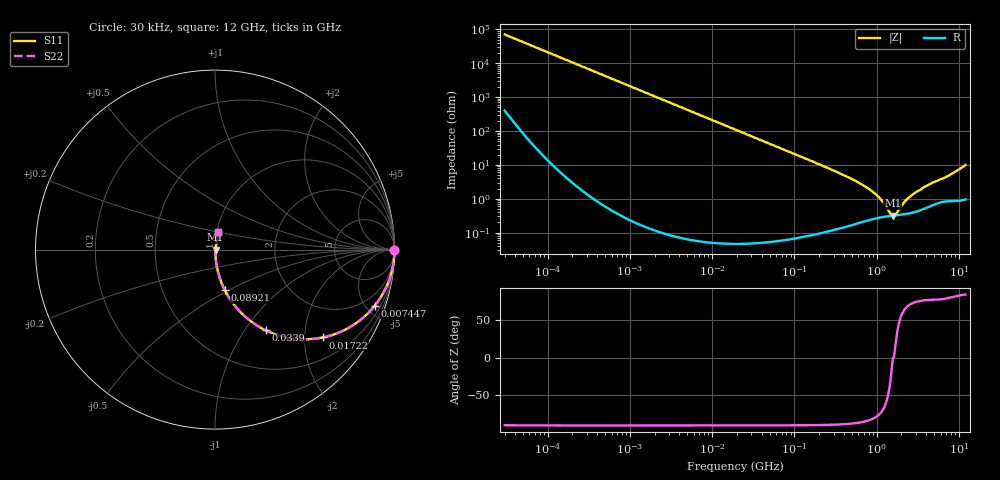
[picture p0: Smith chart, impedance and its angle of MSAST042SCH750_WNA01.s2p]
! MSAST042SCH750_WNA01  S-PARAMETER MODEL  ( General Type )
! Model Generated by TAIYO YUDEN Corporation (http://www.ty-top.com)
! Version 1.0
! TAIYO YUDEN Control No. 150820
! Copyright(c) 2015 TAIYO YUDEN CO.,LTD. All Rights Reserved.
! Product Description (link to TY-COMPAS)
! https://ds.yuden.co.jp/TYCOMPAS/or/detail?pn=MSAST042SCH750JWNA01&u=M
! Products Name : Multilayer Ceramic Capacitors
! Characteristics :
!  Capacitance : 75 pF , Rated Voltage : 25V , TCC : CH / C0H
!  Case Size : 0.4 x 0.2 / 0.016 x 0.008 [mm/inch] , Thickness : 0.2 / 0.008 [mm/inch]
!  (Conditions: Temperature = 25 degC , DC Bias Current/Voltage = 0A / 0V)
! External Node Assignments :
!  1  o---| |---o  2
! GND o---------o GND
! Frequency Range : 0.03MHz  -  12000MHz  [ 401 STEP ]
# MHz S RI R 50
! Freq[MHz].  S11 Real  S11 Imag  S21 Real  S21 Imag  S12 Real  S12 Imag  S22 Real  S22 Imag
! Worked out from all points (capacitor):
!   401 points, 30 kHz to 12 GHz, reference 50 ohm
!   read as one part in series: C = 75 pF near 32 kHz
!   lowest |Z| = 314 mohm at 1.573 GHz (marker M1)
!   series resonance near 1.581 GHz, so ESL is about 140 pH
!   S11 on the Smith chart (normalised r, x): 30 kHz: open; 7.447 MHz: 1.00, -5.70; 17.22 MHz: 1.00, -2.46; 33.9 MHz: 1.00, -1.25; 89.21 MHz: 1.00, -0.47; 12 GHz: 1.02, +0.20
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0.03  1 -0.00141  1e-05 0.00141  1e-05 0.00141  1 -0.00141
0.260295  0.9998 -0.0123  0.000153 0.0123  0.000153 0.0123  0.9998 -0.0123
2.258455  0.9888 -0.1052  0.0112 0.1052  0.0112 0.1052  0.9888 -0.1052
7.447352  0.8903 -0.3124  0.1097 0.3124  0.1097 0.3124  0.8903 -0.3124
11.3258  0.7782 -0.4153  0.2218 0.4153  0.2218 0.4153  0.7782 -0.4153
17.22407  0.6027 -0.4891  0.3973 0.4891  0.3973 0.4891  0.6027 -0.4891
18.97367  0.5556 -0.4967  0.4444 0.4967  0.4444 0.4967  0.5556 -0.4967
33.90345  0.2815 -0.4493  0.7185 0.4493  0.7185 0.4493  0.2815 -0.4493
53.24956  0.1371 -0.3433  0.8629 0.3433  0.8629 0.3433  0.1371 -0.3433
89.2069  0.0538 -0.2242  0.9462 0.2242  0.9462 0.2242  0.0538 -0.2242
164.6252  0.0168 -0.1252  0.9832 0.1252  0.9832 0.1252  0.0168 -0.1252
419.4166  0.00367 -0.0468  0.9963 0.0468  0.9963 0.0468  0.00367 -0.0468
749.4426  0.0027 -0.0218  0.9973 0.0218  0.9973 0.0218  0.0027 -0.0218
1068.55  0.00286 -0.0106  0.9971 0.0106  0.9971 0.0106  0.00286 -0.0106
1215.67  0.00296 -0.00699  0.997 0.00699  0.997 0.00699  0.00296 -0.00699
1428.372  0.00308 -0.0026  0.9969 0.0026  0.9969 0.0026  0.00308 -0.0026
1573.464  0.00313 -9.94e-06  0.9969 9.94e-06  0.9969 9.94e-06  0.00313 -9.94e-06
1733.294  0.00324 0.00155  0.9968 -0.00155  0.9968 -0.00155  0.00324 0.00155
2243.435  0.00359 0.0079  0.9964 -0.0079  0.9964 -0.0079  0.00359 0.0079
2903.719  0.00422 0.0141  0.9958 -0.0141  0.9958 -0.0141  0.00422 0.0141
7640.278  0.0107 0.0478  0.9893 -0.0478  0.9893 -0.0478  0.0107 0.0478
12000  0.0189 0.0959  0.9811 -0.0959  0.9811 -0.0959  0.0189 0.0959
